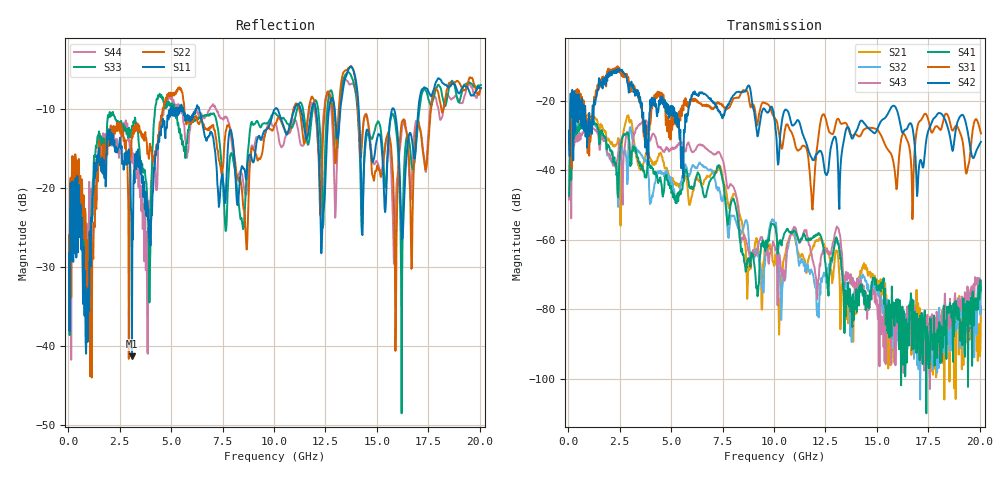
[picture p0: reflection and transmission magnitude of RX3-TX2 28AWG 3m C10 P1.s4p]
! FILE: O:\PROJECTS\SI-2007-05-003 3m Eyemax Qual\XT\FD\RX2-TX1 28AWG 3m C10 P1.s4p
# MHZ S RI R 50.00
! FREQ  S11  S12  S13  S14
!  S21  S22  S23  S24
!  S31  S32  S33  S34
!  S41  S42  S43  S44
!  REAL  IMAG  REAL  IMAG  REAL  IMAG  REAL  IMAG
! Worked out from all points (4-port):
!   801 points, 50 MHz to 20.05 GHz, reference 50 ohm
!   strongest paths, dB at 50 MHz, 5.05 GHz, 10.05 GHz, 15.05 GHz, 20.05 GHz:
!     S42: -28.7, -24.2, -26.5, -27.7, -31.8
!     S31: -28.5, -28.4, -25.2, -28.5, -29.4
!     S41: -47.3, -45.9, -56.3, -73.1, -74.6
!     S43: -48.4, -34.0, -62.3, -82.9, -71.8
!     S32: -47.8, -44.4, -55.5, -75.7, -73.1
!     S21: -46.4, -42.5, -66.7, -72.1, -79.1
!   lowest |S11| = -41.3 dB at 3.1 GHz (marker M1), VSWR 1.02, Z = 50.4 - j0.762 ohm
!   |S11| at or under -10 dB: start of sweep to 4.974 GHz; 6.36 GHz to 10.07 GHz (3.707 GHz wide, 45.1 % of centre); 14.11 GHz to 15.75 GHz (1.635 GHz wide, 10.9 % of centre)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
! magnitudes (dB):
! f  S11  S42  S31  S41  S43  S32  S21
! 50 MHz  -28.3  -28.7  -28.5  -47.3  -48.4  -47.8  -46.4
! 3.1 GHz  -41.3  -15.6  -16.4  -34.6  -34.2  -30.2  -26.7
! 7.325 GHz  -22.5  -22.8  -20.7  -38.5  -34.7  -45.0  -39.0
! 10.3 GHz  -11.0  -30.1  -31.3  -60.1  -65.9  -71.9  -77.0
! 10.88 GHz  -11.2  -27.0  -29.4  -57.9  -57.5  -57.9  -58.2
! 16.2 GHz  -25.3  -28.6  -30.5  -84.2  -85.5  -92.1  -79.6
! 20.05 GHz  -7.4  -31.8  -29.4  -74.6  -71.8  -73.1  -79.1
